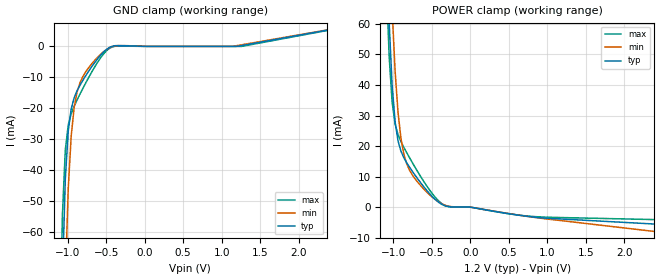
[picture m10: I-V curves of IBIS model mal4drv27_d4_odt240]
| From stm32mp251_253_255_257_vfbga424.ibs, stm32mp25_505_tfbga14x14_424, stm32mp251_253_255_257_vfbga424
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[Model] mal4drv27_d4_odt240
Model_type   Input
Polarity   Non-Inverting
Enable   Active-High
C_comp   1.733pF   1.669pF   1.738pF
C_comp_power_clamp   855.396fF   825.093fF   856.566fF
C_comp_gnd_clamp 768.141fF   766.457fF   774.301fF
Vinh = 720.000mV
Vinl = 605.000mV
[Model Spec]
D_overshoot_ampl_h 0.24 NA   NA
D_overshoot_ampl_l 0.24 NA   NA
D_overshoot_area_l 300.000m NA   NA
D_overshoot_area_h 300.000m NA   NA
[Receiver Thresholds]
Vth = 663.000mV
Vth_min = 630.000mV
Vth_max = 696.000mV
Vinh_ac = 68.000mV
Vinh_dc = 68.000mV
Vinl_ac = -68.000mV
Vinl_dc = -68.000mV
Tslew_ac = 5.000ns
Threshold_sensitivity = 0.5
Reference_supply Power_clamp_ref
[Temperature Range]   25.000   125.000   -40.000
[Voltage Range]   1.200V   1.140V   1.260V
[GND Clamp Reference]   0.00V   0.00V   0.00V
[C Comp Corner]
| variable   typ   min   max
C_comp 1.733pF   1.669pF   1.738pF
C_comp_pullup 856.566fF   825.093fF   855.396fF
C_comp_pulldown 768.141fF   766.457fF   774.301fF
[POWER Clamp Reference]   1.200V   1.140V   1.260V
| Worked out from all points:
|   GND clamp passes 1 mA (typ) near -0.50 V on its own axis
|   POWER clamp passes 1 mA (typ) near -0.38 V on its own axis
[GND Clamp]
-1.184V   -312.2mA   -369.6mA   -285.4mA
-1.107V   -131.8mA   -188.4mA   -102.9mA
-1.069V   -75.44mA   -122.6mA   -54.97mA
-1.031V   -43.02mA   -75.73mA   -33.58mA
-992.7mV  -27.38mA   -46.03mA   -25.46mA
-954.6mV  -20.28mA   -29.05mA   -21.8mA
-916.4mV  -16.67mA   -19.84mA   -19.41mA
-878.2mV  -14.37mA   -14.78mA   -17.37mA
-801.8mV  -10.94mA   -9.721mA   -13.57mA
-496.4mV  -998uA     -1.032mA   -1.422mA
1.184V    82.45nA    187.2uA    4.395nA
2.367V    5.243mA    5.321mA    5.133mA
[Power Clamp]
-1.167V   168.4mA    203.6mA    152.5mA
-1.091V   89.58mA    124.1mA    74.72mA
-1.053V   60.34mA    91.41mA    49.31mA
-1.015V   39.97mA    64.74mA    34.45mA
-976.4mV  27.99mA    44.71mA    27.27mA
-938.2mV  21.71mA    31.04mA    23.73mA
-900mV    18.31mA    22.45mA    21.44mA
-823.6mV  14.45mA    14.07mA    17.76mA
-747.3mV  11.54mA    10.32mA    14.35mA
-365.4mV  824.3uA    1.012mA    1.044mA
818.2mV   -3.269mA   -3.33mA    -3.089mA
2.384V    -5.546mA   -7.965mA   -4.1mA
